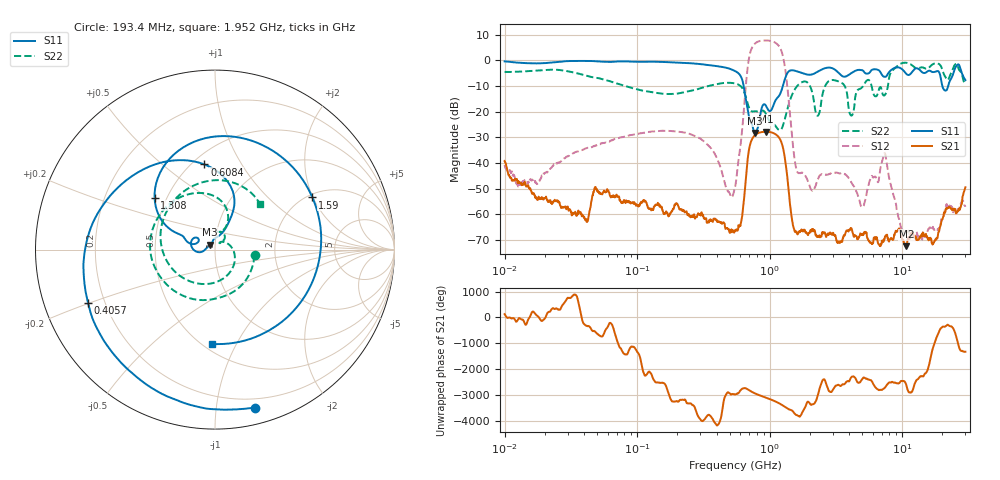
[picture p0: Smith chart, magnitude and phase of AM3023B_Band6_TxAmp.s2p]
# Hz S DB R 50.0
!freq dBS11 angS11 dBS21 angS21 dBS12 angS12 dBS22 angS22
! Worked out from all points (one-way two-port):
!   1601 points, 10 MHz to 30 GHz, reference 50 ohm
!   highest |S21| = -27.83 dB at 940.3 MHz (marker M1); lowest = -72.4 dB at 10.76 GHz (marker M2)
!   lowest |S11| = -28.2 dB at 773.6 MHz (marker M3), VSWR 1.08, Z = 47.4 + j2.68 ohm
!   |S11| at or under -10 dB: 636.5 MHz to 1.258 GHz (621.9 MHz wide, 65.6 % of centre); 20.1 GHz to 22.22 GHz (2.121 GHz wide, 10 % of centre)
!   |S22| runs from -27.2 to -0.9 dB; largest |S21 - S12| = 2.5
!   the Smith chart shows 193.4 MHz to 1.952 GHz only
!   S11 on the Smith chart (normalised r, x): 193.4 MHz: 0.13, -1.28; 405.7 MHz: 0.14, -0.20; 608.4 MHz: 0.57, +0.70; 1.308 GHz: 0.43, +0.31; 1.59 GHz: 2.12, +1.98; 1.952 GHz: 0.55, -0.80
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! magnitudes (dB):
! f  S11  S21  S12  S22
! 10 MHz  -0.4  -39.2  -40.7  -4.5
! 38.04 MHz  -0.2  -59.8  -35.0  -5.5
! 144.7 MHz  -0.6  -56.3  -27.5  -12.8
! 193.4 MHz  -0.8  -56.2  -27.7  -13.1
! 405.7 MHz  -2.3  -62.8  -38.8  -9.2
! 547.7 MHz  -4.2  -66.2  -49.5  -9.0
! 608.4 MHz  -6.4  -63.1  -31.3  -10.2
! 692.9 MHz  -21.2  -35.8  -0.3  -17.9
! 773.6 MHz  -28.2  -29.2  6.5  -19.8
! 940.3 MHz  -17.8  -27.8  7.7  -21.0
! 1.308 GHz  -7.1  -38.7  -3.1  -22.5
! 1.59 GHz  -4.2  -66.6  -42.3  -10.4
! 1.952 GHz  -5.6  -68.1  -47.4  -8.9
! 2.084 GHz  -5.5  -65.7  -50.6  -12.0
! 3.454 GHz  -5.8  -70.6  -44.0  -8.6
! 4.136 GHz  -5.0  -65.4  -47.5  -21.5
! 5.002 GHz  -3.8  -67.6  -57.2  -10.4
! 7.243 GHz  -6.3  -70.5  -37.2  -13.7
! 7.926 GHz  -4.7  -70.3  -45.2  -7.6
! 10.76 GHz  -5.3  -72.4  -67.2  -1.0
! 17.39 GHz  -4.6  -70.9  -65.9  -1.3
! 30 GHz  -7.7  -49.5  -57.0  -9.3
